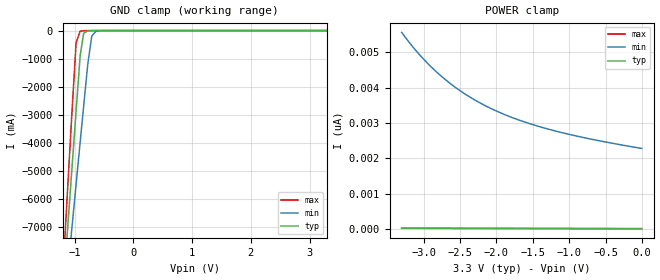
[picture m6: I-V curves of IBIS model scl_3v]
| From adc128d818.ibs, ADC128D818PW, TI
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[Model] scl_3v
Model_type Input
Vinh = 2.31V
Vinl = 0.99V
C_comp   0.51pF   0.46pF   0.60pF
[Voltage Range]   3.3V   3.0V   3.6V
[Temperature Range]   25.0   125.0   -40.0
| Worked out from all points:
|   GND clamp passes 1 mA (typ) near -0.67 V on its own axis
[GND Clamp]
-3.3V     -70.44A    -56.24A    -86.49A
-1.171V   -8.642A    -9.836A    -7.656A
-1.102V   -6.616A    -8.311A    -5.079A
-1.043V   -4.887A    -7.006A    -2.881A
-973.5mV  -2.882A    -5.489A    -436.1mA
-904.2mV  -891.7mA   -3.983A    -21.01mA
-844.8mV  -98.65mA   -2.699A    -4.034mA
-775.5mV  -9.682mA   -1.21A     -1.083mA
-706.2mV  -1.603mA   -192.7mA   -225.4uA
-636.9mV  -323.1uA   -27.96mA   -32.85uA
-438.9mV  -1.555uA   -177.5uA   -28.52nA
3.293V    10.94pA    0A         9.88pA
[POWER Clamp]
-3.3V     24.82pA    5.565nA    20.79pA
-3.161V   23.94pA    5.192nA    20.38pA
-3.033V   23.16pA    4.884nA    19.99pA
-2.765V   21.69pA    4.344nA    19.19pA
-2.627V   20.98pA    4.11nA     18.77pA
-2.458V   20.17pA    3.861nA    18.27pA
-2.3V     19.44pA    3.658nA    17.79pA
-2.092V   18.54pA    3.43nA     17.17pA
-1.696V   16.94pA    3.09nA     15.98pA
-1.261V   15.31pA    2.813nA    14.67pA
-696.3mV  13.32pA    2.544nA    12.98pA
-3.3mV    10.97pA    2.281nA    10.9pA
